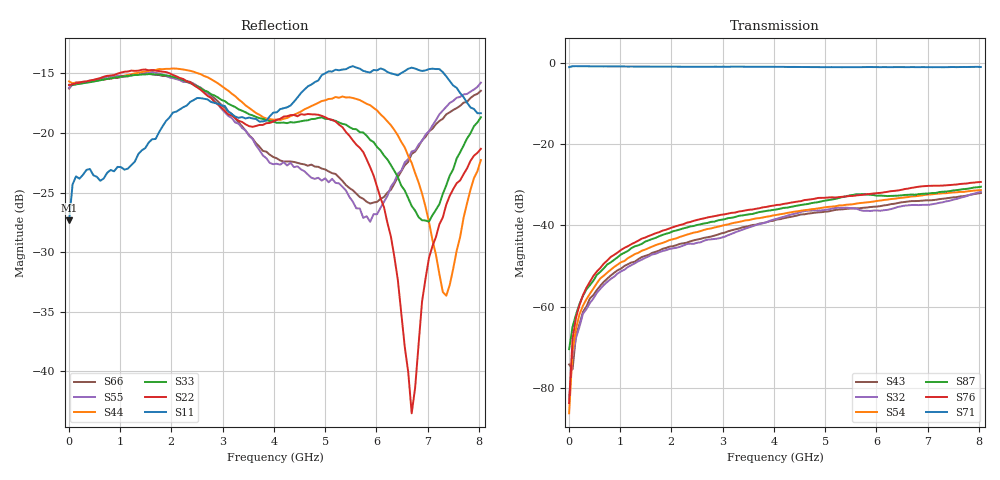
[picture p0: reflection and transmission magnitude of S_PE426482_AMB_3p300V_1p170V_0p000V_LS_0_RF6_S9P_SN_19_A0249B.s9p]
! Device ID: PE426482
! File Path: z:\PE426482\Final Char Data\room\AMB\3p300\LS_0_RF6\PE426482_AMB_3p300V_1p170V_0p000V_LS_0_RF6_S9P_SN_19_A0249B.s9p
! Serial: 19
! Lot: A0249B
! Temp: AMB
! VDD: 3.300
! VSS: 0.000
! Control_Hi: 1.170
! Control_Lo: 0.000
! Logic State: LS_0_RF6
! Port 1:
! Port 2:
! Port 3:
! Port 4:
! Port 5:
! Port 6:
! Port 7:
! Port 8:
! Port 9:
! ThroughPath:1-7
! IDD: 0.0001087638
! ISS/IDD2: 5.48e-008
! IDMM3/IDD3: -2.357e-007
! Comment:
#  Hz  S  RI  R  50
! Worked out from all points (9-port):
!   120 points, 10 MHz to 8.037 GHz, reference 50 ohm
!   strongest paths, dB at 10 MHz, 2.034 GHz, 4.057 GHz, 6.08 GHz, 8.037 GHz:
!     S71: -1.0, -0.9, -1.0, -1.0, -1.0
!     S76: -83.7, -40.4, -35.0, -32.0, -29.3
!     S87: -70.4, -41.4, -36.0, -32.6, -30.5
!     S54: -86.2, -43.4, -37.4, -33.9, -31.3
!     S32: -82.7, -45.6, -38.4, -36.4, -31.7
!     S43: -74.2, -45.1, -38.5, -35.2, -32.0
!   lowest |S11| = -27.3 dB at 10 MHz (marker M1), VSWR 1.09, Z = 53.7 - j2.54 ohm
!   |S11| at or under -10 dB: start of sweep to end of sweep
